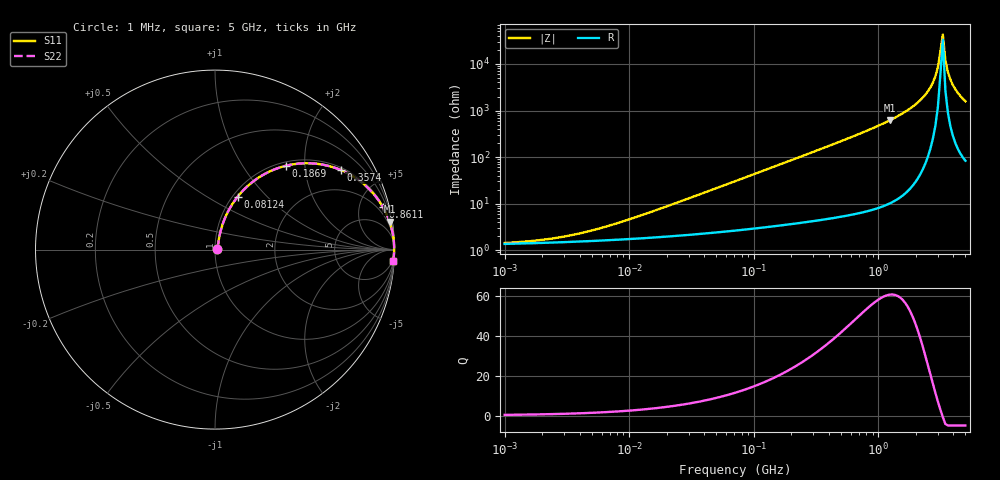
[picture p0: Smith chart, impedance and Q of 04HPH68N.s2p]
# MHz S MA R 50
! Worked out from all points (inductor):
!   185 points, 1 MHz to 5 GHz, reference 50 ohm
!   read as one part in series: L = 68 nH near 12.75 MHz
!   highest Q = 60.8 at 1.247 GHz (marker M1), where L = 79.6 nH
!   self-resonance near 3.147 GHz
!   S11 on the Smith chart (normalised r, x): 1 MHz: 1.03, +0.01; 81.24 MHz: 1.06, +0.69; 186.9 MHz: 1.07, +1.60; 357.4 MHz: 1.09, +3.09; 861.1 MHz: 1.14, +7.91; 5 GHz: 3, -32
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1  0.01418 17.1  0.9865 -0.2  0.9865 -0.2  0.01418 17.1
2.19661  0.01706 32.3  0.9856 -0.5  0.9856 -0.5  0.01706 32.3
4.19948  0.02336 48.1  0.9846 -1.0  0.9846 -1.0  0.02336 48.1
17.6357  0.07609 71.5  0.9785 -4.2  0.9785 -4.2  0.07609 71.5
70.7107  0.2836 68.6  0.9345 -16.4  0.9345 -16.4  0.2836 68.6
81.2446  0.3212 66.8  0.922 -18.7  0.922 -18.7  0.3212 66.8
186.918  0.6125 49.7  0.7637 -37.7  0.7637 -37.7  0.6125 49.7
296.948  0.7757 37.3  0.606 -50.8  0.606 -50.8  0.7757 37.3
357.35  0.8286 32.4  0.536 -55.9  0.536 -55.9  0.8286 32.4
861.097  0.9653 14.1  0.2441 -74.8  0.2441 -74.8  0.9653 14.1
1247.03  0.9849 9.1  0.1578 -80.0  0.1578 -80.0  0.9849 9.1
1981.11  0.9956 4.3  0.07426 -84.5  0.07426 -84.5  0.9956 4.3
2276.24  0.9971 3.0  0.05263 -85.3  0.05263 -85.3  0.9971 3.0
2615.33  0.998 1.8  0.03195 -85.4  0.03195 -85.4  0.998 1.8
2869.02  0.9982 1.1  0.01853 -84.0  0.01853 -84.0  0.9982 1.1
3004.94  0.9983 0.7  0.01192 -81.3  0.01192 -81.3  0.9983 0.7
3296.42  0.9982 -0.1  0.002328 39.0  0.002328 39.0  0.9982 -0.1
3452.59  0.9981 -0.5  0.008317 76.3  0.008317 76.3  0.9981 -0.5
3616.17  0.9979 -0.8  0.01488 81.4  0.01488 81.4  0.9979 -0.8
3787.49  0.9976 -1.2  0.02152 83.1  0.02152 83.1  0.9976 -1.2
4154.87  0.9969 -2.0  0.03497 84.0  0.03497 84.0  0.9969 -2.0
5000  0.9947 -3.6  0.06281 83.4  0.06281 83.4  0.9947 -3.6
